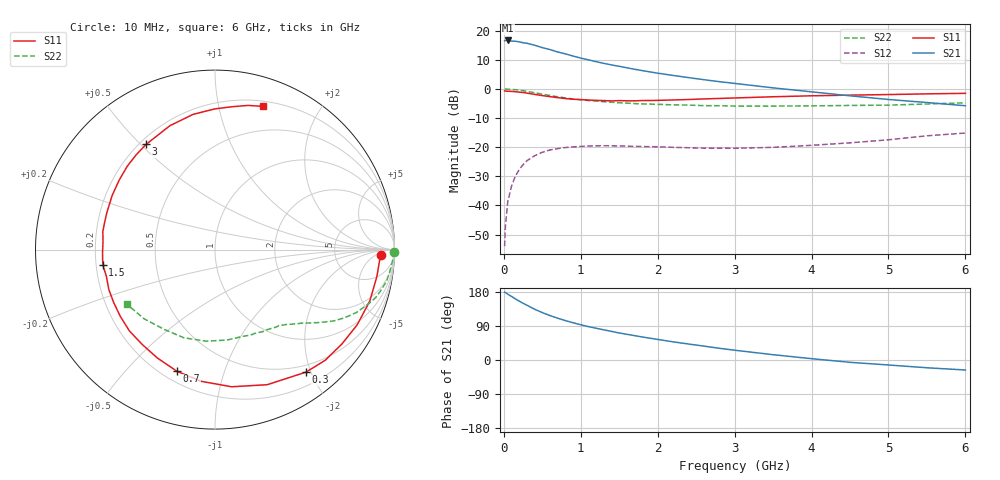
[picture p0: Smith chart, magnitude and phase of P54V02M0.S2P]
! SIEMENS Small Signal Semiconductors
! BFP183
! Si NPN RF Bipolar Junction Transistor in SOT143
! VCE = 4 V  IC = 2 mA
! Common Emitter S-Parameters:  March  1996
# GHz  S  MA  R  50
!  f  S11  S21  S12  S22
! GHz  MAG  ANG  MAG  ANG  MAG  ANG  MAG  ANG
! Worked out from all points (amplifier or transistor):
!   36 points, 10 MHz to 6 GHz, reference 50 ohm
!   highest |S21| = 16.7 dB at 50 MHz (marker M1)
!   |S21| within 3 dB of that: start of sweep to 579 MHz
!   unconditionally stable (mu >= 1): 2.131 GHz to 5.804 GHz
!   at 250 MHz: K = 0.12, MSG = 20.9 dB, |S12| = -26.0 dB
!   at 1.4 GHz: K = 0.67, MSG = 13.9 dB, |S12| = -19.5 dB
!   at 6 GHz: K = 0.97, MSG = 4.7 dB, |S12| = -15.1 dB
!   S11 on the Smith chart (normalised r, x): 10 MHz: 22, -10; 300 MHz: 0.39, -1.93; 700 MHz: 0.26, -0.70; 1.5 GHz: 0.23, -0.06; 3 GHz: 0.23, +0.52; 6 GHz: 0.25, +1.36
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0.01  0.9258 -2.0  6.736 179.0  0.002 89.6  0.9991 -0.7
0.02  0.9192 -3.7  6.795 178.1  0.0043 87.7  0.9931 -1.4
0.05  0.9144 -9.4  6.805 173.7  0.0114 87.0  0.9915 -3.5
0.1  0.9089 -18.4  6.622 167.7  0.0215 78.5  0.9819 -7.0
0.15  0.8962 -27.9  6.607 161.3  0.0319 73.8  0.9719 -10.4
0.2  0.8812 -36.6  6.436 155.4  0.0412 69.5  0.9541 -13.5
0.3  0.8504 -53.4  6.096 144.6  0.0586 60.4  0.9097 -19.2
0.4  0.8069 -68.9  5.638 133.9  0.0715 52.5  0.8623 -24.0
0.5  0.7698 -83.1  5.121 125.1  0.0818 45.1  0.815 -27.8
0.6  0.7378 -96.0  4.74 117.2  0.0897 39.6  0.7732 -30.9
0.7  0.7101 -107.4  4.321 110.3  0.0945 34.8  0.7339 -33.3
0.9  0.6662 -127.5  3.676 98.3  0.1013 27.1  0.6733 -37.3
1.1  0.6457 -144.7  3.162 88.0  0.1051 21.4  0.6332 -40.3
1.3  0.6321 -159.3  2.751 79.5  0.106 16.9  0.6046 -43.2
1.5  0.6311 -172.3  2.449 71.3  0.1051 14.2  0.5799 -45.8
1.8  0.633 170.8  2.067 60.7  0.1029 11.5  0.5538 -50.1
2.2  0.6475 152.2  1.708 47.9  0.0996 10.1  0.5335 -56.4
3  0.7008 123.2  1.246 25.8  0.0958 13.8  0.5083 -71.7
3.5  0.7346 110.0  1.045 14.0  0.0995 18.2  0.5082 -82.5
4.5  0.7841 90.0  0.763 -6.1  0.1189 24.0  0.521 -109.4
5.5  0.8241 77.1  0.585 -20.5  0.1569 24.5  0.5521 -135.8
6  0.8415 71.5  0.515 -26.4  0.1753 21.2  0.5784 -148.4
